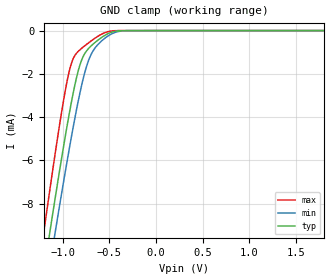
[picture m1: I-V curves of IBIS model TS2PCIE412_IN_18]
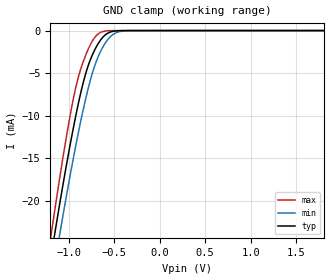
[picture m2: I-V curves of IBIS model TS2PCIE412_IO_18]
| TEXAS INSTRUMENTS INCORPORATED
| Standard Linear and Logic Group
| IBIS Model of TS2PCIE412
| 4-Channel PCI Express 2:1 Multiplexer Switch for PCIe Data Applications
| This file contains package information for the following:
|  qfn 42-pin (RUA) package as [Component] TS2PCIE412_RUA
| This device can be powered at the following Vccs:
|  1.8 volt Vcc
| This file provides unique models under the [Model Selector] for each Vcc.
| For operation at a specific Vcc, select the appropriate model after each
| [Model Selector] keyword.
[IBIS Ver]   3.2
[Comment char]  |_char
[File Name]   ts2pcie412.ibs
[File Rev]   1.1 | x_die
[Date]   October 7, 2008
[Source]   Data created from TI-SPICE simulations at TI-SLL.
[Notes]   The following is an IBIS list for the TS2PCIE412.
   Please contact sllibis@ti.com with questions and
   comments concerning SLL IBIS models.
   - FILE REV HISTORY
   - 1.1 Release IBIS File on 10/08/08
   - Power clamp data deleted was deleted as there is no
   power-clamp diode.
[Disclaimer] Property of Texas Instruments Incorporated.  Unauthorized
   reproduction and/or distribution is strictly prohibited.
   This product is protected under copyright law.
   Created  2008, (C) Copyright  2008, Texas Instruments
   Incorporated, All Rights Reserved
   UNLESS THERE IS A SIGNED, WRITTEN AGREEMENT TO THE
   CONTRARY, TEXAS INSTRUMENTS (TI) IS PROVIDING THE IBIS
   MODELS  AND WITHOUT ANY WARRANTY, EXPRESSED OR
   IMPLIED.  TI assumes no liability for:
   1) the accuracy of the IBIS models provided to your
   company;
   2) the proper functioning of these IBIS Models in your
   design or for any resulting applications; or
   3) infringement of patents, copyrights or intellectual
   property rights resulting from your use of these IBIS
   models.
   TI provides IBIS Models as a service to our customers.
   You and your company shall not distribute, sell or give
   these models to anyone else without prior written
   permission from TI.
   TI reserves the right to make changes to our products or
   to discontinue any semiconductor product or service
   without notice, and advises our customers to obtain the
   latest version of relevant information to verify, before
   placing orders, that the information being relied on is
   current.
   Please be aware that your receipt and use of the IBIS
   information provided shall serve as acceptance of these
   terms and conditions.  If you do not accept these terms,
   you should return or destroy the IBIS models and any
   other accompanying information immediately.
| Component TS2PCIE412_RUA 42-PIN QFN
[Component]   TS2PCIE412_RUA
[Manufacturer]   Texas Instruments, Inc.
[Package]
|   typ   min   max
R_pkg   1.024e-01   6.263e-02   1.372e-01
L_pkg   2.245e-09   1.300e-09   3.156e-09
C_pkg   2.642e-13   1.816e-13   3.573e-13
[Pin]   signal_name   model_name   R_pin   L_pin   C_pin
1   GND   GND   1.358e-01   3.026e-09   2.905e-13
2   A0   TS2PCIE412_IO_18   1.290e-01   2.862e-09   3.263e-13
3   A1   TS2PCIE412_IO_18   1.158e-01   2.549e-09   3.115e-13
4   GND   GND   1.029e-01   2.247e-09   2.774e-13
5   VCC   POWER   9.101e-02   1.968e-09   2.469e-13
6   A2   TS2PCIE412_IO_18   8.034e-02   1.720e-09   2.222e-13
7   A3   TS2PCIE412_IO_18   7.122e-02   1.509e-09   1.996e-13
8   VCC   POWER   6.616e-02   1.393e-09   1.889e-13
9   SEL   TS2PCIE412_IN_18   6.303e-02   1.321e-09   1.857e-13
10   GND   GND   6.449e-02   1.355e-09   1.889e-13
11   A4   TS2PCIE412_IO_18   7.023e-02   1.486e-09   2.008e-13
12   A5   TS2PCIE412_IO_18   7.899e-02   1.688e-09   2.192e-13
13   VCC   POWER   8.950e-02   1.933e-09   2.417e-13
14   GND   GND   1.007e-01   2.195e-09   2.662e-13
15   A6   TS2PCIE412_IO_18   1.120e-01   2.460e-09   2.982e-13
16   A7   TS2PCIE412_IO_18   1.254e-01   2.775e-09   3.215e-13
17   GND   GND   1.345e-01   2.996e-09   2.925e-13
18   VCC   POWER   1.365e-01   3.140e-09   3.562e-13
19   GND   GND   1.292e-01   2.864e-09   2.970e-13
20   VCC   POWER   1.292e-01   2.862e-09   2.969e-13
21   GND   GND   1.366e-01   3.137e-09   3.562e-13
22   7B2   TS2PCIE412_IO_18   1.348e-01   2.997e-09   3.023e-13
23   6B2   TS2PCIE412_IO_18   1.211e-01   2.668e-09   3.116e-13
24   5B2   TS2PCIE412_IO_18   1.100e-01   2.405e-09   2.864e-13
25   4B2   TS2PCIE412_IO_18   9.879e-02   2.142e-09   2.577e-13
26   7B1   TS2PCIE412_IO_18   8.940e-02   1.921e-09   2.377e-13
27   6B1   TS2PCIE412_IO_18   7.884e-02   1.675e-09   2.186e-13
28   5B1   TS2PCIE412_IO_18   6.993e-02   1.468e-09   2.000e-13
29   4B1   TS2PCIE412_IO_18   6.414e-02   1.334e-09   1.876e-13
30   VCC   POWER   6.263e-02   1.300e-09   1.816e-13
31   3B2   TS2PCIE412_IO_18   6.461e-02   1.345e-09   1.858e-13
32   2B2   TS2PCIE412_IO_18   7.083e-02   1.489e-09   2.017e-13
33   1B2   TS2PCIE412_IO_18   7.997e-02   1.701e-09   2.210e-13
34   0B2   TS2PCIE412_IO_18   9.067e-02   1.951e-09   2.406e-13
35   3B1   TS2PCIE412_IO_18   1.002e-01   2.174e-09   2.611e-13
36   2B1   TS2PCIE412_IO_18   1.115e-01   2.440e-09   2.898e-13
37   1B1   TS2PCIE412_IO_18   1.225e-01   2.700e-09   3.136e-13
38   0B1   TS2PCIE412_IO_18   1.356e-01   3.015e-09   3.026e-13
39   GND   GND   1.372e-01   3.154e-09   3.573e-13
40   VCC   POWER   1.299e-01   2.879e-09   2.983e-13
41   GND   GND   1.299e-01   2.881e-09   2.983e-13
42   VCC   POWER   1.372e-01   3.156e-09   3.567e-13
[Series Switch Groups]
| Function Group States
On  1 /   | A0-A7->0B1-7B1 SEL LOW
On  2 /   | A0-A7->0B2-7B2 SEL HIGH
[Series Pin Mapping]   pin_2   model_name   function_table_group
2   38   TS2PCIE412_IO_18_S   1
3   37   TS2PCIE412_IO_18_S   1
6   36   TS2PCIE412_IO_18_S   1
7   35   TS2PCIE412_IO_18_S   1
11   29   TS2PCIE412_IO_18_S   1
12   28   TS2PCIE412_IO_18_S   1
15   27   TS2PCIE412_IO_18_S   1
16   26   TS2PCIE412_IO_18_S   1
2   34   TS2PCIE412_IO_18_S   2
3   33   TS2PCIE412_IO_18_S   2
6   32   TS2PCIE412_IO_18_S   2
7   31   TS2PCIE412_IO_18_S   2
11   25   TS2PCIE412_IO_18_S   2
12   24   TS2PCIE412_IO_18_S   2
15   23   TS2PCIE412_IO_18_S   2
16   22   TS2PCIE412_IO_18_S   2
| Model TS2PCIE412_IO
[Model]   TS2PCIE412_IO_18_S
Model_type  Series_switch
| variable   typ   min   max
C_comp   0   0   0
[Temperature Range]   40   100   -40
| Ambient temperature   25   85   -40
[Voltage range]   1.8   1.65   1.95
[On]
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[Off]
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| Models and submodels in the file (3): TS2PCIE412_IN_18 (Input), TS2PCIE412_IO_18_S (Series_switch), TS2PCIE412_IO_18 (Terminator)
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| Model TS2PCIE412_IN
[Model]   TS2PCIE412_IN_18
Model_type  Input
Vinl=0.63
Vinh=1.17
| variable   typ   min   max
C_comp   0.78pF   0.65pF   0.98pF
[Temperature Range]   40   100   -40
| Ambient temperature   25   85   -40
[Voltage range]   1.8   1.65   1.95
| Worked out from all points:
|   GND clamp passes 1 mA (typ) near -0.75 V on its own axis
[GND Clamp]
| TS2PCIE412_IN_18
|   Voltage   I(typ)   I(min)   I(max)
-1.8V     -28.54mA   -29.3mA    -28.18mA
-1.215V   -11.48mA   -12.93mA   -9.691mA
-1.185V   -10.64mA   -12.12mA   -8.778mA
-1.14V    -9.378mA   -10.91mA   -7.425mA
-1.075V   -7.593mA   -9.178mA   -5.523mA
-965mV    -4.71mA    -6.346mA   -2.612mA
-895mV    -3.055mA   -4.644mA   -1.377mA
-820mV    -1.661mA   -2.986mA   -907.9uA
-745mV    -945.9uA   -1.671mA   -641.4uA
-615mV    -419.6uA   -613uA     -245.2uA
-350mV    -3.145uA   -13.45uA   -158.1nA
1.8V      791.1pA    34.39nA    8.363pA
| Model TS2PCIE412_IO_S
[Model]   TS2PCIE412_IO_18
Model_type  Terminator
| variable   typ   min   max
C_comp   1.14pF   0.99pF   1.34pF
| C_tri-state   1.14pF   0.99pF   1.34pF
[Temperature Range]   40   100   -40
| Ambient temperature   25   85   -40
[Voltage range]   1.8   1.65   1.95
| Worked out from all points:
|   GND clamp passes 1 mA (typ) near -0.64 V on its own axis
[GND Clamp]
| TS2PCIE412_IO_18
|   Voltage   I(typ)   I(min)   I(max)
-1.8V     -71.88mA   -74.47mA   -73.12mA
-1.2V     -27.15mA   -30.68mA   -24.67mA
-1.18V    -25.81mA   -29.36mA   -23.21mA
-1.145V   -23.49mA   -27.07mA   -20.7mA
-1.085V   -19.63mA   -23.25mA   -16.54mA
-975mV    -13.02mA   -16.61mA   -9.574mA
-890mV    -8.477mA   -11.9mA    -5.392mA
-785mV    -4.151mA   -6.834mA   -2.211mA
-655mV    -1.216mA   -2.603mA   -258.9uA
-535mV    -152.3uA   -663.3uA   -8.734uA
-405mV    -5.344uA   -56.02uA   -51.69nA
1.8V      749.9pA    33.76nA    10.73pA
